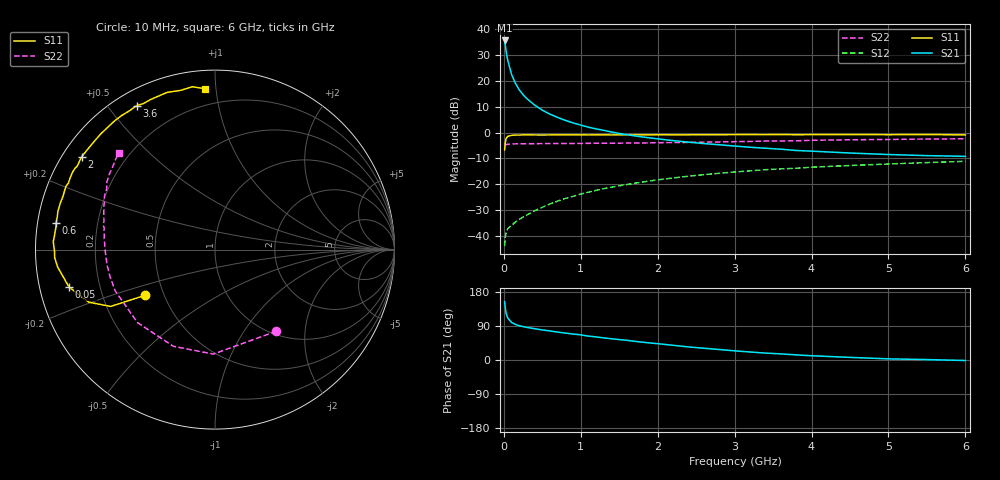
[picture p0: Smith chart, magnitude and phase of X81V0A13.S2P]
! SIEMENS Small Signal Semiconductors
! BFP136W
! Si NPN RF Bipolar Junction Transistor in SOT343
! VCE = 1 V  IC = 130 mA
! Common Emitter S-Parameters:  September  1994
# GHz  S  MA  R  50
!  f  S11  S21  S12  S22
! GHz  MAG  ANG  MAG  ANG  MAG  ANG  MAG  ANG
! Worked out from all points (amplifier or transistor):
!   40 points, 10 MHz to 6 GHz, reference 50 ohm
!   highest |S21| = 35.5 dB at 10 MHz (marker M1)
!   |S21| within 3 dB of that: start of sweep to 24.55 MHz
!   unconditionally stable (mu >= 1): 347.1 MHz to end of sweep
!   at 200 MHz: K = 0.82, MSG = 25.0 dB, |S12| = -33.6 dB
!   at 1.5 GHz: K = 1.17, MAG = 7.6 dB, |S12| = -20.6 dB
!   at 6 GHz: K = 1.06, MAG = -0.5 dB, |S12| = -11.1 dB
!   S11 on the Smith chart (normalised r, x): 10 MHz: 0.39, -0.26; 50 MHz: 0.09, -0.13; 600 MHz: 0.05, +0.08; 2 GHz: 0.05, +0.31; 3.6 GHz: 0.06, +0.59; 6 GHz: 0.10, +0.94
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0.01  0.4639 -146.8  59.87 153.9  0.0064 57.5  0.5691 -53.0
0.02  0.6617 -151.4  47.3 135.0  0.0097 47.0  0.5822 -90.9
0.03  0.7619 -157.4  37.16 123.3  0.0117 41.2  0.5866 -113.3
0.05  0.8397 -165.6  24.98 111.0  0.0139 33.2  0.5931 -136.7
0.1  0.8822 -173.7  13.26 99.1  0.0161 36.3  0.6018 -157.5
0.15  0.8949 -177.3  8.92 93.9  0.0187 40.4  0.6035 -165.2
0.2  0.8941 -179.4  6.676 90.5  0.021 44.6  0.6056 -169.3
0.25  0.8987 178.6  5.379 88.0  0.0234 48.1  0.6075 -172.0
0.3  0.9022 177.2  4.497 86.1  0.0255 50.9  0.6077 -173.9
0.4  0.8968 174.3  3.385 82.4  0.0309 55.5  0.6093 -176.4
0.5  0.895 172.0  2.702 79.3  0.036 57.8  0.6106 -178.3
0.6  0.8975 170.5  2.258 76.8  0.0418 60.3  0.6115 -179.7
0.8  0.9008 166.4  1.713 71.1  0.0533 62.4  0.614 178.1
1.1  0.8971 160.6  1.266 63.0  0.0705 62.6  0.6183 175.3
1.5  0.8999 154.0  0.959 53.9  0.0938 61.0  0.6233 171.9
2  0.9053 145.1  0.755 43.1  0.122 56.7  0.6372 167.4
2.2  0.9032 141.8  0.698 38.8  0.1326 54.8  0.6386 165.7
3.2  0.9104 124.8  0.52 21.1  0.1819 44.2  0.673 156.1
3.6  0.9132 118.6  0.477 16.1  0.1987 40.1  0.6879 152.5
4.5  0.9157 106.9  0.402 6.9  0.2308 31.1  0.7241 144.3
5.5  0.9161 97.9  0.358 1.1  0.2628 23.1  0.7486 137.7
6  0.8977 93.5  0.347 -1.3  0.2782 18.6  0.7568 134.8
